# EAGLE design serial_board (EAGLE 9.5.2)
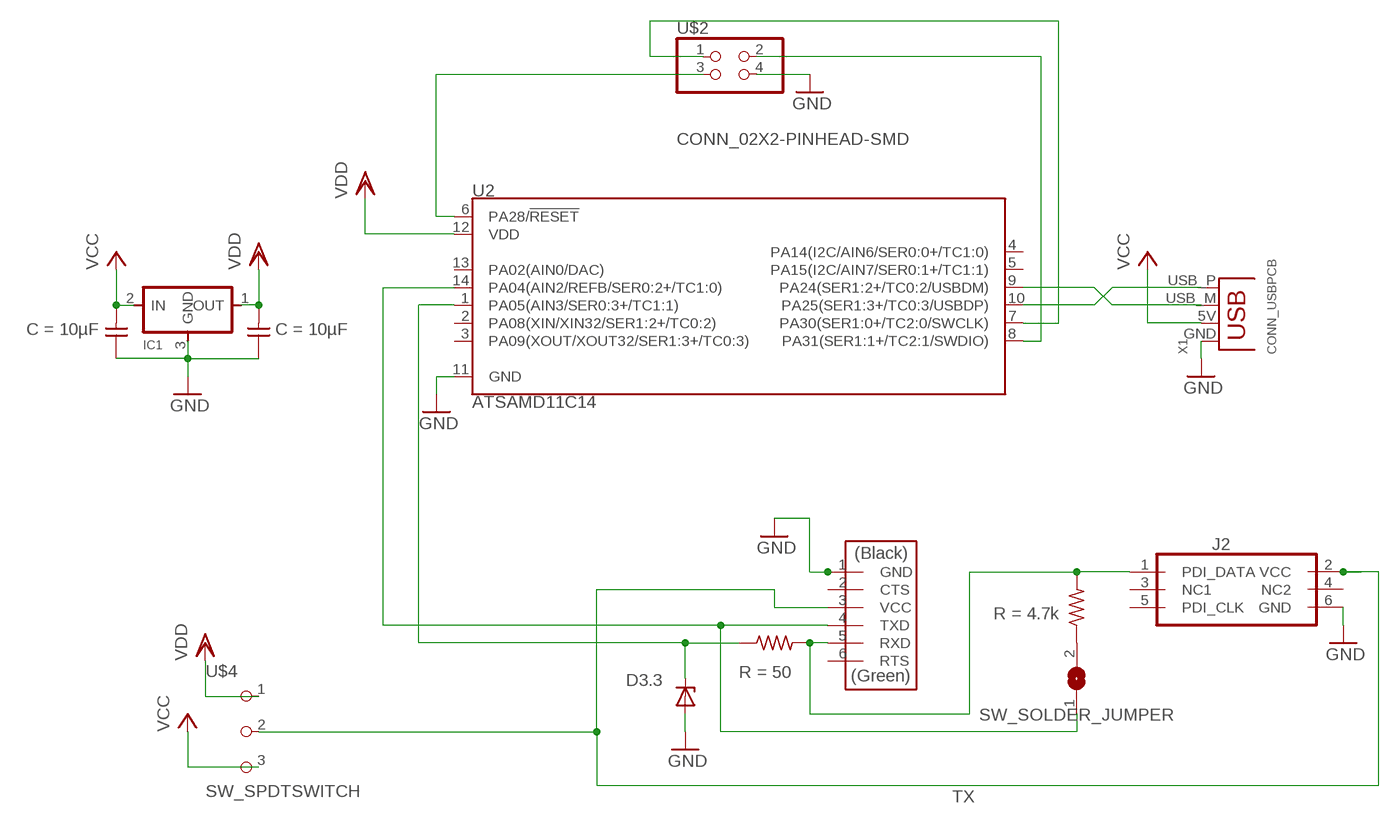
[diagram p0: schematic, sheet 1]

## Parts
C1  CAP_UNPOLARIZEDFAB  [C1206FAB]
C2  CAP_UNPOLARIZEDFAB  [C1206FAB]
D3.3  DIODE_ZENERSOD123  [SOD123]
IC1  VR_REGULATOR-SOT23SOT23  [SOT23]
J2  CONN_03X2_PDIFEMALE_SMD  [PDI_2X3_SMD]
R1  SW_SOLDER_JUMPER  [SJFAB]
R2  R1206FAB  [R1206FAB]
R_SER  R1206FAB  [R1206FAB]
U2  ATSAMD11C14  [SOIC-14]
U$1  CONN_06_FTDI-SMD-HEADER  [1X06SMD]
U$2  CONN_02X2-PINHEAD-SMD  [2X02SMD]
U$4  SW_SPDTSWITCH  [SPDTSWITCH]
X1  CONN_USBPCB  [USB-A-PCB]

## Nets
CLK: U2.7(PA30(SER1:0+/TC2:0/SWCLK)) U$2.1
DIO: U2.8(PA31(SER1:1+/TC2:1/SWDIO)) U$2.2
GND: C1.1 C2.1 D3.3.ANODE IC1.3(GND) J2.6(GND) U2.11(GND) U$1.1(GND) U$2.4 X1.GND
N$1: R1.2 R_SER.1
N$2: U2.9(PA24(SER1:2+/TC0:2/USBDM)) X1.USB_M(D-)
N$3: U2.10(PA25(SER1:3+/TC0:3/USBDP)) X1.USB_P(D+)
RES: U2.6(PA28/!RESET!) U$2.3
RX: D3.3.CATHODE R2.1 U2.1(PA05(AIN3/SER0:3+/TC1:1))
RX_RAW: J2.1(PDI_DATA) R2.2 R_SER.2 U$1.5(RXD)
TX: R1.1 U2.14(PA04(AIN2/REFB/SER0:2+/TC1:0)) U$1.4(TXD)
V_TARGET: J2.2(VCC) U$1.3(VCC) U$4.2
VCC: C2.2 IC1.2(IN) U$4.3 X1.5V(VBUS)
VDD: C1.2 IC1.1(OUT) U2.12(VDD) U$4.1
Unconnected: J2.3(NC1) J2.4(NC2) J2.5(PDI_CLK) U2.2(PA08(XIN/XIN32/SER1:2+/TC0:2)) U2.3(PA09(XOUT/XOUT32/SER1:3+/TC0:3)) U2.4(PA14(I2C/AIN6/SER0:0+/TC1:0)) U2.5(PA15(I2C/AIN7/SER0:1+/TC1:1)) U2.13(PA02(AIN0/DAC)) U$1.2(CTS) U$1.6(RTS)

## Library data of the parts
C1 C2 = fab:CAP_UNPOLARIZED; C: 10µF
D3.3 = fab:DIODE_ZENER: zener diode
IC1 = fab:VR_REGULATOR-SOT23
J2 = fab:CONN_03X2_PDI: Multi connection point. Often used as Generic Header-pin footprint for 0.1 inch spaced/style header connections You can populate with any combo of single row headers, but if you'd like an exact match, check these: Header - 2x3 (Male, 0.1") (PRT-12807) Header - 2x3 (Female, 0.1") (PRT-13010) 2x3 Pin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; PROD_ID: CONN-11290
R1 = fab:SW_SOLDER_JUMPER
R2 = fab:R: Resistor (US Symbol); R: 50
R_SER = fab:R: Resistor (US Symbol); R: 4.7k
U2 = SAMD11C_Mini_Breakout:ATSAMD11C14: Atmel SAM D11 SMART ARM-Based Microcontroller The Atmel® | SMART™ SAM D11 is a series of low-power microcontrollers using the 32-bit ARM® Cortex®-M0+ processor, and ranging from 14- to 24-pins with 16KB Flash and 4KB of SRAM. The SAM D11 devices operate at a maximum frequency of 48MHz and reach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
U$1 = fab:CONN_06_FTDI-SMD-HEADER
U$2 = fab:CONN_02X2-PINHEAD-SMD
U$4 = fab:SW_SPDTSWITCH
X1 = fab:CONN_USB: USB Connectors USB-B-PTH is fully proven SKU : PRT-00139 USB-miniB is fully proven SKU : PRT-00587 USB-A-PCB is untested. USB-A-H is throughly reviewed, but untested. Spark Fun Electronics SKU : PRT-00437 USB-B-SMT is throughly reviewed, but untested. Needs silkscreen touching up. USB-A-S has not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

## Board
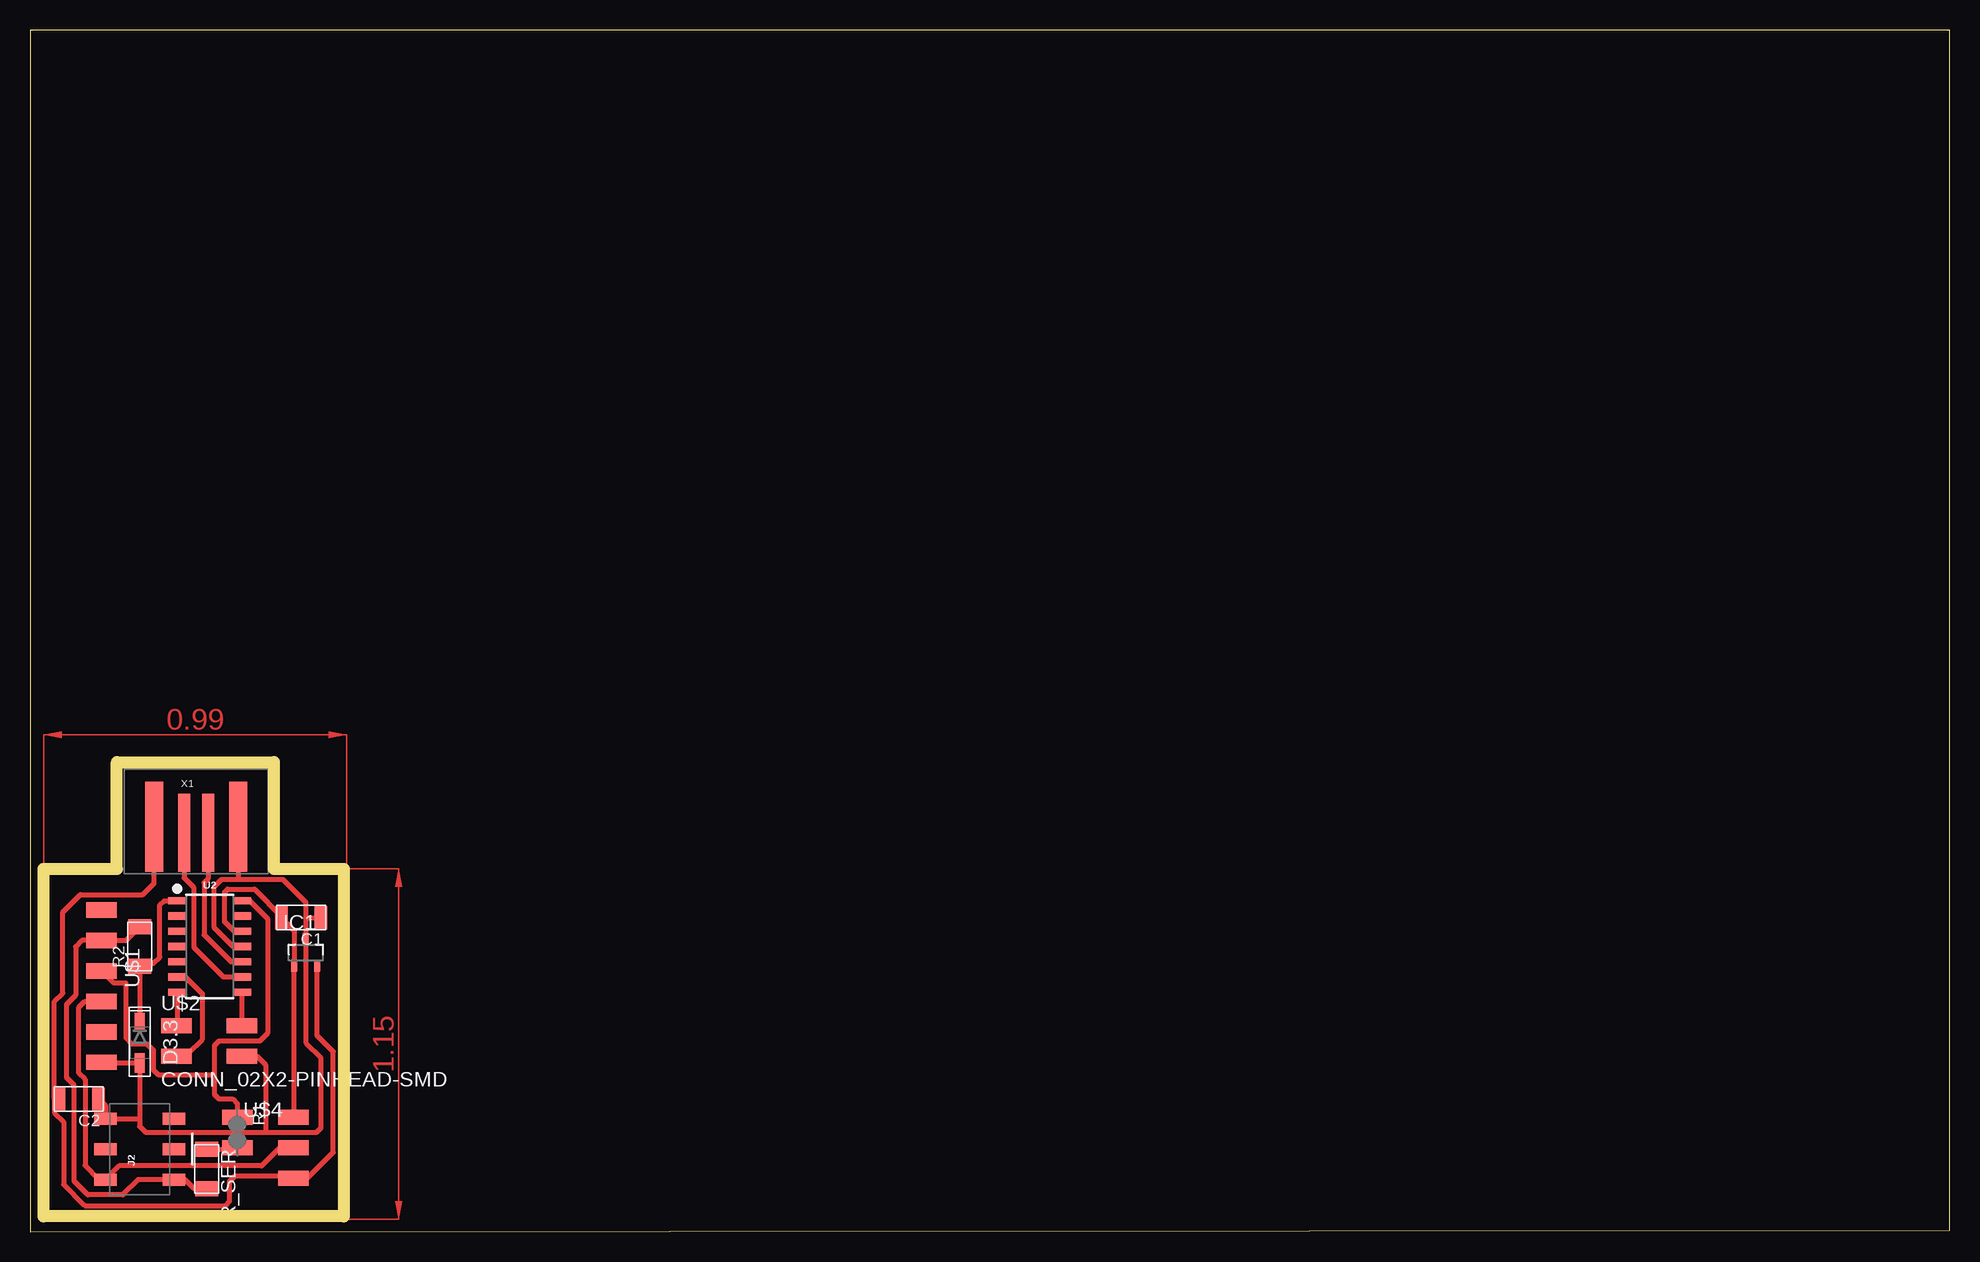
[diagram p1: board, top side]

Size 160 x 100.13 mm. Coordinates in mm from the lower left corner, seen from the top.
Outline: 0,0 160,0.13 160,100.13 0,100.13 0,0
Copper layers (1*16): Top 0.035mm / dielectric 1.5mm / Bottom 0.035mm
Design rules "default *": minimum track width 16mil, minimum drill 0.35mm, track to track 16mil, track to pad 16mil, pad to pad 16mil, via to via 8mil, smd to smd 6mil, copper to edge 40mil, drill to drill 6mil, minimum pad ring 10mil, minimum via ring 8mil, stop-mask expansion 4mil, vias tented up to drill 0mil, thermal gap 10mil
Milling: 8 lines

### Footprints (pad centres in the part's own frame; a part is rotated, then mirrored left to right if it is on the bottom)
C1206FAB = smd 1.016 x 1.905: 1 -1.651,0; 2 1.651,0
SOD123 = smd 1.6 x 0.8: ANODE 1.7,0; CATHODE -1.7,0
SOT23 = smd 0.508 x 1.016: 1 -0.95,-1.1; 2 0.95,-1.1; 3 0,1.1
PDI_2X3_SMD = smd 1.02 x 1.9: 1 -2.54,-2.85; 2 -2.54,2.85; 3 0,-2.85; 4 0,2.85; 5 2.54,-2.85; 6 2.54,2.85
SJFAB = smd 1.27 x 2.54: 1 -0.635,0; 2 1.905,0
R1206FAB = smd 1.27 x 1.905: 1 -1.651,0; 2 1.651,0
SOIC-14 = smd 0.6 x 1.5: 1 -3.81,-2.7; 2 -2.54,-2.7; 3 -1.27,-2.7; 4 0,-2.7; 5 1.27,-2.7; 6 2.54,-2.7; 7 3.81,-2.7; 8 3.81,2.7; 9 2.54,2.7; 10 1.27,2.7; 11 0,2.7; 12 -1.27,2.7; 13 -2.54,2.7; 14 -3.81,2.7
1X06SMD = smd 2.54 x 1.27: 1 0,6.35; 2 0,3.81; 3 0,1.27; 4 0,-1.27; 5 0,-3.81; 6 0,-6.35
2X02SMD = smd 2.54 x 1.27: 1 -2.54,1.27; 2 2.92,1.27; 3 -2.54,-1.27; 4 2.92,-1.27
SPDTSWITCH = smd 2.54 x 1.27: 1 0.38,2.54; 2 0.38,0; 3 0.38,-2.54
USB-A-PCB = smd 7.5 x 1.5: 5V -0.2,-3.5; GND -0.2,3.5 | smd 6.5 x 1: USB_M 0.3,-1; USB_P 0.3,1

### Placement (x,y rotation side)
C1  22.61,26.16 180 top
C2  4.06,11.05 180 top
D3.3  9.14,15.75 270 top
IC1  22.99,23.24 0 top
J2  9.14,6.86 90 top
R1  17.27,8.89 270 top
R2  9.14,23.75 90 top
R_SER  14.73,5.21 270 top
U2  14.99,23.75 270 top
U$1  5.97,20.45 180 top
U$2  14.73,15.88 0 top
U$4  21.59,6.98 0 top
X1  13.84,33.53 270 top

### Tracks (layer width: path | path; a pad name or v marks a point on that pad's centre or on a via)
CLK
  Top 0.406: U$2.1 12.29,17.24 U2.7
DIO
  Top 0.406: U$2.2 17.69,17.18 U2.8
GND
  Top 0.406: U2.11 16.92,23.75 15.37,25.3 15.37,28.74 15.97,29.34 17.32,29.34 | X1.GND 17.34,29.36 17.32,29.34 | 9.14,9.4 D3.3.ANODE 6.02,14.05 U$1.1 | 9.14,9.4 J2.6 6.29,10.47 C2.1 | 9.14,9.4 9.14,8.76 9.65,8.26 19.68,8.26 | 17.32,29.34 21.08,29.34 22.99,27.43 22.99,26.04 | U$2.4 18.92,14.61 19.68,13.84 19.68,8.26 | 19.68,8.26 23.88,8.26 24.26,8.64 24.26,14.48 22.99,15.75 IC1.3 22.99,26.04 | 22.99,26.04 23.11,26.16 C1.1
N$1
  Top 0.406: R_SER.1 16.93,6.86 R1.2
N$2
  Top 0.406: X1.USB_M 12.84,29.46 13.67,28.63 13.67,23.67 16.13,21.21 U2.9
N$3
  Top 0.406: U2.10 16.76,22.48 14.51,24.73 14.51,29.08 14.84,29.41 X1.USB_P
RES
  Top 0.406: U2.6 12.97,21.2 14.38,19.79 14.38,16.03 13.21,14.86 12.45,14.86 U$2.3
RX
  Top 0.406: D3.3.CATHODE R2.1 9.4,22.35 10.29,22.35 10.79,22.86 10.83,22.86 10.83,27.22 11.18,27.56 U2.1
RX_RAW
  Top 0.406: R2.2 8,24.26 U$1.5 4.32,24.26 3.81,23.75 3.81,19.68 3.05,18.92 3.05,12.83 3.68,12.19 3.68,4.2 4.83,3.05 7.75,3.05 9.02,4.32 J2.1 12.93,4.32 13.69,3.56 R_SER.2
TX
  Top 0.406: R1.1 17.27,10.67 16.89,11.05 15.75,11.05 15.37,11.43 15.37,13.21 | 15.37,13.21 15.37,15.49 15.75,15.88 19.15,15.88 19.81,16.54 19.81,26.07 18.33,27.56 U2.14 | U$1.4 6.99,20.7 8,20.7 8,16.13 8.51,15.62 9.78,15.62 10.29,15.11 10.29,13.46 10.67,13.08 15.24,13.08 15.37,13.21
V_TARGET
  Top 0.406: U$4.2 20.83,6.98 19.3,5.46 7.44,5.46 J2.2 5.79,4.32 4.6,5.51 4.6,12.68 4.06,13.21 4.06,18.67 4.57,19.18 U$1.3
VCC
  Top 0.406: 2.03,11.05 2.03,19.18 2.73,19.88 2.73,26.61 4.19,28.07 9.4,28.07 10.34,29.01 X1.5V | 2.03,11.05 2.03,9.91 2.79,9.14 2.79,3.94 4.57,2.16 16.29,2.16 16.64,2.5 16.64,4.19 17.09,4.64 21.97,4.64 U$4.3 23.11,4.44 25.27,6.6 25.27,14.99 23.94,16.32 IC1.2 | C2.2 2.03,11.05
VDD
  Top 0.406: 18.19,25.02 U2.12 17.02,25.02 16.23,25.81 16.23,28.29 16.46,28.52 18.72,28.52 20.95,26.29 C1.2 22.04,25.08 IC1.1 21.97,22.07 U$4.1
(copper drawn outside any net)
  shapes: Top area x2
